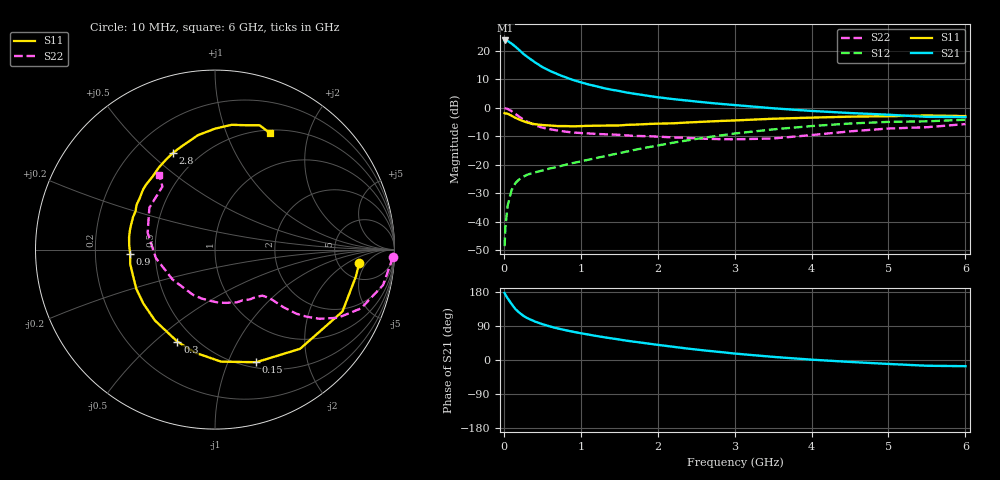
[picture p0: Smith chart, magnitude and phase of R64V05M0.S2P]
! SIEMENS Small Signal Semiconductors
! BFR193
! Si NPN RF Bipolar Junction Transistor in SOT23
! VCE = 4 V  IC = 5 mA
! Common Emitter S-Parameters:  May  1996
# GHz  S  MA  R  50
!  f  S11  S21  S12  S22
! GHz  MAG  ANG  MAG  ANG  MAG  ANG  MAG  ANG
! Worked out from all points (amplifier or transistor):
!   36 points, 10 MHz to 6 GHz, reference 50 ohm
!   highest |S21| = 23.7 dB at 20 MHz (marker M1)
!   |S21| within 3 dB of that: start of sweep to 184.8 MHz
!   unconditionally stable (mu >= 1): 896 MHz to 1.994 GHz
!   at 250 MHz: K = 0.43, MSG = 21.7 dB, |S12| = -24.2 dB
!   at 1.4 GHz: K = 1.07, MAG = 9.9 dB, |S12| = -16.5 dB
!   at 6 GHz: K = 0.96, MSG = 0.5 dB, |S12| = -4.2 dB
!   lowest NFmin = 1.20 dB at 450 MHz
!   S11 on the Smith chart (normalised r, x): 10 MHz: 7.80, -3.45; 150 MHz: 0.56, -1.27; 300 MHz: 0.40, -0.59; 900 MHz: 0.36, -0.02; 2.8 GHz: 0.36, +0.59; 6 GHz: 0.54, +1.44
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0.01  0.8067 -5.5  15.19 176.8  0.0037 85.6  0.9917 -2.4
0.02  0.7991 -10.8  15.34 172.7  0.0081 83.6  0.981 -4.8
0.05  0.7896 -25.9  15.03 162.7  0.0193 76.9  0.9571 -11.9
0.1  0.7281 -49.4  13.53 147.8  0.0356 66.6  0.8774 -21.9
0.15  0.6682 -69.9  11.96 134.4  0.0475 58.7  0.7835 -29.0
0.2  0.625 -86.9  10.41 125.0  0.0554 54.1  0.6984 -33.5
0.25  0.5857 -100.5  9.019 117.3  0.0614 50.2  0.6308 -36.3
0.3  0.554 -112.2  7.983 111.0  0.0665 48.5  0.5776 -38.2
0.4  0.5177 -130.3  6.403 101.9  0.0732 47.3  0.4982 -40.1
0.5  0.4993 -143.2  5.232 94.6  0.0792 47.9  0.45 -40.8
0.6  0.4899 -153.6  4.47 88.5  0.0861 48.9  0.4216 -41.3
0.7  0.4791 -162.9  3.913 83.3  0.092 50.7  0.4001 -42.2
0.9  0.4732 -176.8  3.099 74.6  0.1075 53.6  0.3684 -44.2
1.1  0.4834 172.0  2.588 67.1  0.1226 56.1  0.3554 -47.7
1.3  0.488 162.6  2.224 60.2  0.1405 57.7  0.344 -51.4
1.6  0.5033 150.3  1.859 50.8  0.1709 59.1  0.3281 -59.0
2.2  0.5356 130.4  1.429 34.9  0.2442 57.3  0.3032 -78.3
2.8  0.5877 113.5  1.182 21.3  0.3255 51.3  0.2825 -105.2
3.5  0.6445 98.5  0.984 8.3  0.4186 40.6  0.2895 -145.0
4.5  0.7015 82.4  0.812 -5.1  0.5317 23.9  0.3868 166.0
5.5  0.736 70.3  0.696 -15.2  0.5803 6.7  0.4574 129.8
6  0.7174 64.6  0.691 -16.3  0.6189 1.7  0.5192 126.8
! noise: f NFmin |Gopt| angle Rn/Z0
0.45  1.2  0.26  102  0.14
0.9  1.25  0.38  145  0.12
1.8  2.05  0.56  -161  0.12
